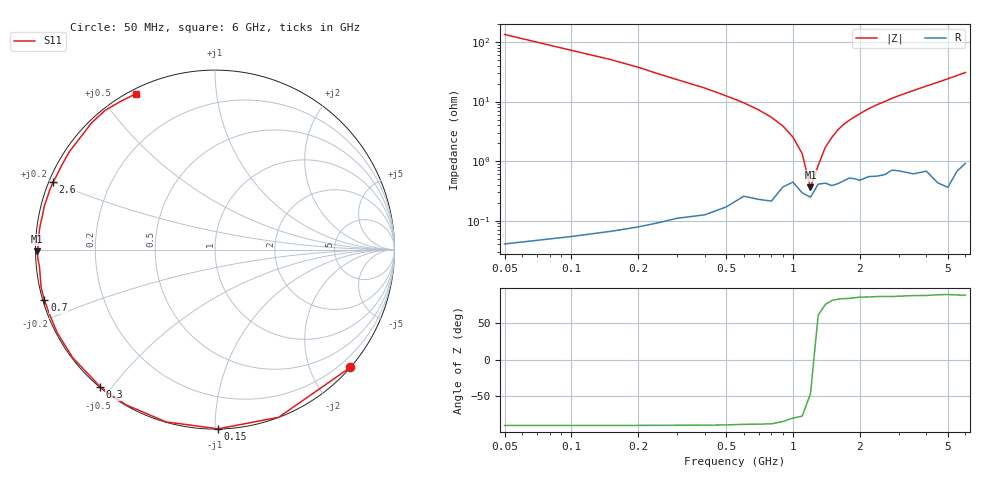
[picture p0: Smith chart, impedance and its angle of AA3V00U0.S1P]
! Infineon Technologies  Discrete & RF Semiconductors
! BBY66-02W
! Si Tuning Diode in SCD-80
! VR = 3 V
! S-Parameters:  June  2000
# GHz  S  MA  R  50
!  f  S11
! GHz  MAG  ANG
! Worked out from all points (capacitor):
!   34 points, 50 MHz to 6 GHz, reference 50 ohm
!   read as one part to ground: C = 21.8 pF near 50 MHz
!   lowest |Z| = 361 mohm at 1.2 GHz (marker M1)
!   series resonance near 1.226 GHz, so ESL is about 770 pH
!   S11 on the Smith chart (normalised r, x): 50 MHz: 0.00, -2.67; 150 MHz: 0.00, -1.02; 300 MHz: 0.00, -0.47; 700 MHz: 0.00, -0.14; 2.6 GHz: 0.01, +0.20; 6 GHz: 0.02, +0.62
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0.05  0.9998 -41.0
0.1  0.9993 -69.2
0.15  0.9987 -89.0
0.2  0.998 -105.9
0.25  0.9972 -120.1
0.3  0.9964 -129.9
0.4  0.9955 -142.7
0.5  0.9936 -152.0
0.6  0.9901 -158.4
0.7  0.9911 -163.5
0.8  0.9916 -167.6
0.9  0.9855 -171.1
1  0.9824 -174.3
1.1  0.9883 -177.0
1.2  0.9901 -179.4
1.4  0.9831 176.2
1.6  0.9834 172.3
1.7  0.9815 170.5
2  0.9814 165.8
2.4  0.9785 159.9
2.6  0.9774 157.3
3  0.9744 151.9
3.5  0.9779 145.9
4  0.9763 140.0
4.5  0.9854 134.3
5  0.9883 128.4
5.5  0.9793 122.6
6  0.9738 116.8
